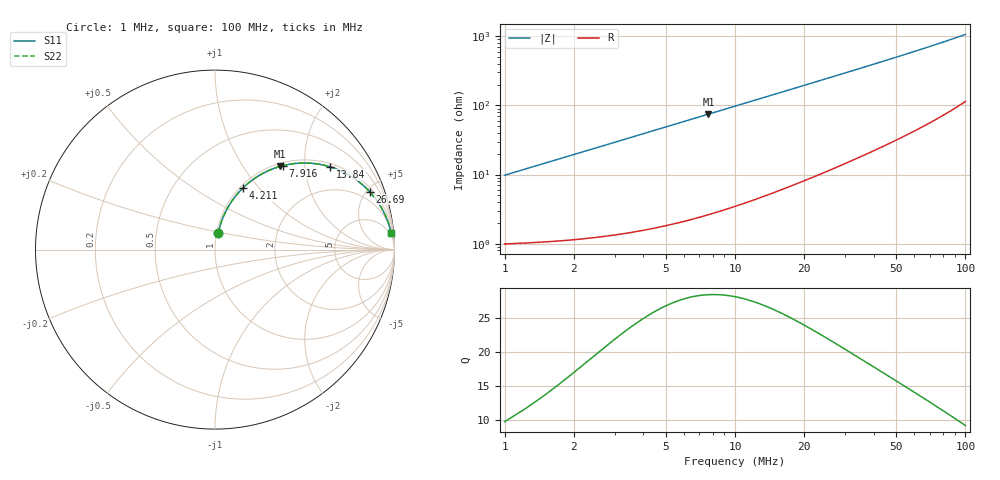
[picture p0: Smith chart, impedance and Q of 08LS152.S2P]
! Coilcraft 0805LS-152 Chip Inductor
! 18 September 2002
# MHZ S MA R 50
!Freq  MagS11  AngS11  MagS21  AngS21  MagS12  AngS12  MagS22  AngS22
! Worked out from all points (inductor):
!   402 points, 1 MHz to 100 MHz, reference 50 ohm
!   read as one part in series: L = 1.55 uH near 1.494 MHz
!   highest Q = 28.4 at 7.669 MHz (marker M1), where L = 1.55 uH
!   S11 on the Smith chart (normalised r, x): 1 MHz: 1.02, +0.19; 4.211 MHz: 1.03, +0.82; 7.916 MHz: 1.05, +1.54; 13.84 MHz: 1.10, +2.70; 26.69 MHz: 1.24, +5.22; 100 MHz: 3, +21
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1  0.09648 78.7  0.9856 -5.5  0.9856 -5.5  0.09648 78.7
1.247  0.1198 78.3  0.9828 -6.9  0.9828 -6.9  0.1198 78.3
1.988  0.1883 75.8  0.9711 -10.8  0.9711 -10.8  0.1883 75.8
2.482  0.2325 73.7  0.9608 -13.4  0.9608 -13.4  0.2325 73.7
3.223  0.296 70.3  0.9422 -17.2  0.9422 -17.2  0.296 70.3
4.211  0.3745 65.8  0.9126 -22.0  0.9126 -22.0  0.3745 65.8
4.952  0.4284 62.5  0.8877 -25.3  0.8877 -25.3  0.4284 62.5
5.693  0.4778 59.4  0.8613 -28.5  0.8613 -28.5  0.4778 59.4
7.669  0.5888 51.9  0.7879 -36.0  0.7879 -36.0  0.5888 51.9
7.916  0.6007 51.1  0.7787 -36.9  0.7787 -36.9  0.6007 51.1
9.398  0.6639 46.4  0.7248 -41.6  0.7248 -41.6  0.6639 46.4
10.88  0.7149 42.3  0.674 -45.6  0.674 -45.6  0.7149 42.3
13.844  0.7896 35.8  0.5847 -52.1  0.5847 -52.1  0.7896 35.8
17.549  0.849 29.7  0.4956 -58.0  0.4956 -58.0  0.849 29.7
21.748  0.8903 24.7  0.4188 -62.8  0.4188 -62.8  0.8903 24.7
26.688  0.9198 20.6  0.3519 -66.8  0.3519 -66.8  0.9198 20.6
34.098  0.945 16.3  0.2819 -70.7  0.2819 -70.7  0.945 16.3
42.002  0.9597 13.3  0.2312 -73.4  0.2312 -73.4  0.9597 13.3
50.647  0.9692 11.1  0.1923 -75.3  0.1923 -75.3  0.9692 11.1
67.196  0.9787 8.2  0.1439 -77.4  0.1439 -77.4  0.9787 8.2
83.745  0.9833 6.5  0.1135 -78.3  0.1135 -78.3  0.9833 6.5
100  0.9858 5.3  0.09279 -78.5  0.09279 -78.5  0.9858 5.3
